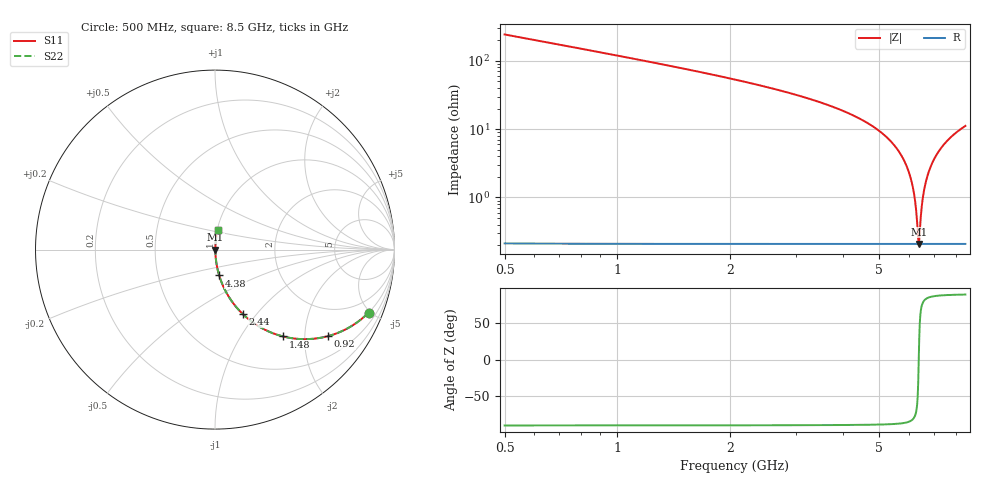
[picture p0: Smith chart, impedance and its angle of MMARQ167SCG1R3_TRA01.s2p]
! MMARQ167SCG1R3_TRA01  S-PARAMETER MODEL  ( General Type )
! Model Generated by TAIYO YUDEN Corporation (http://www.ty-top.com)
! Version 1.0
! TAIYO YUDEN Control No. 160201
! Copyright(c) 2016 TAIYO YUDEN CO.,LTD. All Rights Reserved.
! Product Description (link to TY-COMPAS)
! https://ds.yuden.co.jp/TYCOMPAS/or/detail?pn=MMARQ167SCG1R3BTRA01&u=M
! Products Name : Multilayer Ceramic Capacitors
! Characteristics :
!  Capacitance : 1.3 pF , Rated Voltage : 250V , TCC : CG / C0G
!  Case Size : 1.6 x 0.8 / 0.063 x 0.031 [mm/inch] , Thickness : 0.7 / 0.028 [mm/inch]
!  (Conditions: Temperature = 25 degC , DC Bias Current/Voltage = 0A / 0V)
! External Node Assignments :
!  1  o---| |---o  2
! GND o---------o GND
! Frequency Range : 500MHz  -  8500MHz  [ 401 STEP ]
# MHz S RI R 50
! Freq[MHz].  S11 Real  S11 Imag  S21 Real  S21 Imag  S12 Real  S12 Imag  S22 Real  S22 Imag
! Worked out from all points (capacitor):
!   401 points, 500 MHz to 8.5 GHz, reference 50 ohm
!   read as one part in series: C = 1.3 pF near 540 MHz
!   lowest |Z| = 208 mohm at 6.38 GHz (marker M1)
!   series resonance near 6.381 GHz, so ESL is about 480 pH
!   S11 on the Smith chart (normalised r, x): 500 MHz: 1.00, -4.87; 920 MHz: 1.00, -2.61; 1.48 GHz: 1.00, -1.57; 2.44 GHz: 1.00, -0.86; 4.38 GHz: 1.00, -0.30; 8.5 GHz: 1.00, +0.22
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500  0.8553 -0.3514  0.1447 0.3514  0.1447 0.3514  0.8553 -0.3514
920  0.6291 -0.4822  0.3709 0.4822  0.3709 0.4822  0.6291 -0.4822
1480  0.3802 -0.4841  0.6198 0.4841  0.6198 0.4841  0.3802 -0.4841
1840  0.2719 -0.4432  0.7281 0.4432  0.7281 0.4432  0.2719 -0.4432
2440  0.1563 -0.3607  0.8437 0.3607  0.8437 0.3607  0.1563 -0.3607
3180  0.0789 -0.266  0.9211 0.266  0.9211 0.266  0.0789 -0.266
4380  0.0233 -0.1441  0.9767 0.1441  0.9767 0.1441  0.0233 -0.1441
4500  0.0203 -0.1337  0.9797 0.1337  0.9797 0.1337  0.0203 -0.1337
5300  0.00715 -0.071  0.9928 0.071  0.9928 0.071  0.00715 -0.071
5840  0.00323 -0.0338  0.9968 0.0338  0.9968 0.0338  0.00323 -0.0338
6020  0.00257 -0.0222  0.9974 0.0222  0.9974 0.0222  0.00257 -0.0222
6160  0.00226 -0.0135  0.9977 0.0135  0.9977 0.0135  0.00226 -0.0135
6260  0.00213 -0.0073  0.9979 0.0073  0.9979 0.0073  0.00213 -0.0073
6340  0.00209 -0.00245  0.9979 0.00245  0.9979 0.00245  0.00209 -0.00245
6380  0.00208 -4.23e-05  0.9979 4.23e-05  0.9979 4.23e-05  0.00208 -4.23e-05
6420  0.00208 0.00235  0.9979 -0.00235  0.9979 -0.00235  0.00208 0.00235
6520  0.00215 0.00825  0.9979 -0.00825  0.9979 -0.00825  0.00215 0.00825
6660  0.00235 0.0164  0.9977 -0.0164  0.9977 -0.0164  0.00235 0.0164
6880  0.00291 0.0288  0.9971 -0.0288  0.9971 -0.0288  0.00291 0.0288
7180  0.00412 0.0451  0.9959 -0.0451  0.9959 -0.0451  0.00412 0.0451
7740  0.00758 0.0739  0.9924 -0.0739  0.9924 -0.0739  0.00758 0.0739
8500  0.0143 0.1097  0.9857 -0.1097  0.9857 -0.1097  0.0143 0.1097
